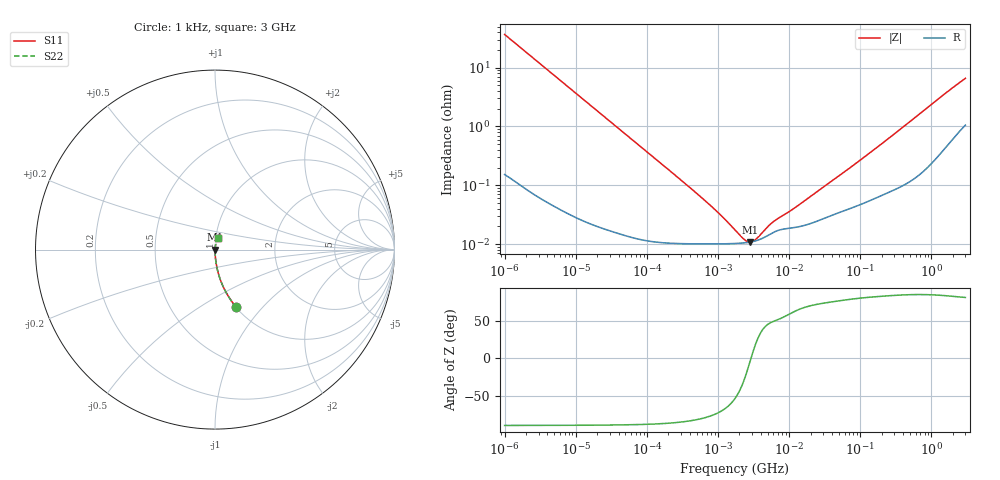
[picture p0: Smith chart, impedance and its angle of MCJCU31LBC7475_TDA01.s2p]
! MCJCU31LBC7475_TDA01  S-PARAMETER MODEL  ( Standard Model )
! Model Generated by TAIYO YUDEN Corporation (http://www.ty-top.com)
! Version 1.0
! TAIYO YUDEN Control No. 220601
! Copyright(c) 2016 TAIYO YUDEN CO.,LTD. All Rights Reserved.
! Product Description (link to TY-COMPAS)
! https://ds.yuden.co.jp/TYCOMPAS/or/detail?pn=MCJCU31LBC7475KTDA01&u=M
! Products Name : Multilayer Ceramic Capacitors
! Characteristics :
!  Capacitance : 4.7 [uF] , Rated Voltage : 50 [V] , TCC : X7S
!  Case Size : 3.2 x 1.6 / 0.126 x 0.063 [mm/inch] , Thickness : 1.6 / 0.063 [mm/inch]
!  (Conditions: Temperature = 25 [degC] , DC Bias Voltage = 0 [V])
! External Node Assignments :
!  1  o---| |---o  2
! GND o---------o GND
! Frequency Range : 1kHz  -  3GHz  [ 401 STEP ]
# MHZ S RI R 50
! Freq[MHz].  S11 Real  S11 Imag  S21 Real  S21 Imag  S12 Real  S12 Imag  S22 Real  S22 Imag
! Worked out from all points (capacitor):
!   401 points, 1 kHz to 3 GHz, reference 50 ohm
!   read as one part in series: C = 4.33 uF near 1.077 kHz
!   lowest |Z| = 10.9 mohm at 2.812 MHz (marker M1)
!   series resonance near 2.912 MHz, so ESL is about 690 pH
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0.001  0.1196 -0.3224  0.8804 0.3224  0.8804 0.3224  0.1196 -0.3224
0.001685  0.0462 -0.2077  0.9538 0.2077  0.9538 0.2077  0.0462 -0.2077
0.00306  0.0148 -0.1184  0.9852 0.1184  0.9852 0.1184  0.0148 -0.1184
0.005768  0.00446 -0.0636  0.9955 0.0636  0.9955 0.0636  0.00446 -0.0636
0.01216  0.00118 -0.0303  0.9988 0.0303  0.9988 0.0303  0.00118 -0.0303
0.147855  0.000113 -0.00251  0.9999 0.00251  0.9999 0.00251  0.000113 -0.00251
0.734727  0.000101 -0.000476  0.9999 0.000476  0.9999 0.000476  0.000101 -0.000476
1.149317  0.000101 -0.000275  0.9999 0.000275  0.9999 0.000275  0.000101 -0.000275
1.732051  0.000103 -0.00014  0.9999 0.00014  0.9999 0.00014  0.000103 -0.00014
2.334012  0.000105 -5.78e-05  0.9999 5.78e-05  0.9999 5.78e-05  0.000105 -5.78e-05
2.610246  0.000107 -2.84e-05  0.9999 2.84e-05  0.9999 2.84e-05  0.000107 -2.84e-05
2.812335  0.000108 -9e-06  0.9999 9e-06  0.9999 9e-06  0.000108 -9e-06
3.03007  0.00011 1.04e-05  0.9999 -1.04e-05  0.9999 -1.04e-05  0.00011 1.04e-05
3.388684  0.000114 3.96e-05  0.9999 -3.96e-05  0.9999 -3.96e-05  0.000114 3.96e-05
5.106836  0.000142 0.000145  0.9999 -0.000145  0.9999 -0.000145  0.000142 0.000145
6.153411  0.000161 0.000187  0.9998 -0.000187  0.9998 -0.000187  0.000161 0.000187
11.1738  0.00019 0.000341  0.9998 -0.000341  0.9998 -0.000341  0.00019 0.000341
21.06097  0.000229 0.00064  0.9998 -0.00064  0.9998 -0.00064  0.000229 0.00064
74.82276  0.000414 0.00202  0.9996 -0.00202  0.9996 -0.00202  0.000414 0.00202
256.0921  0.000806 0.00636  0.9992 -0.00636  0.9992 -0.00636  0.000806 0.00636
1533.384  0.00543 0.0353  0.9946 -0.0353  0.9946 -0.0353  0.00543 0.0353
3000  0.0145 0.0634  0.9855 -0.0634  0.9855 -0.0634  0.0145 0.0634
